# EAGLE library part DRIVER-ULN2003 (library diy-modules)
7-Channel Darlington NPN Transistor Module based on ULN2003 chip More details available here: https://www.elecrow.com/wiki/index.php?title=ULN2003_Stepper_Motor_Driver ULN2003 datasheet available here: http://www.ti.com/lit/ds/slrs027o/slrs027o.pdf Click here to find device on ebay.com Note: There are many variants. Search for the proper version.
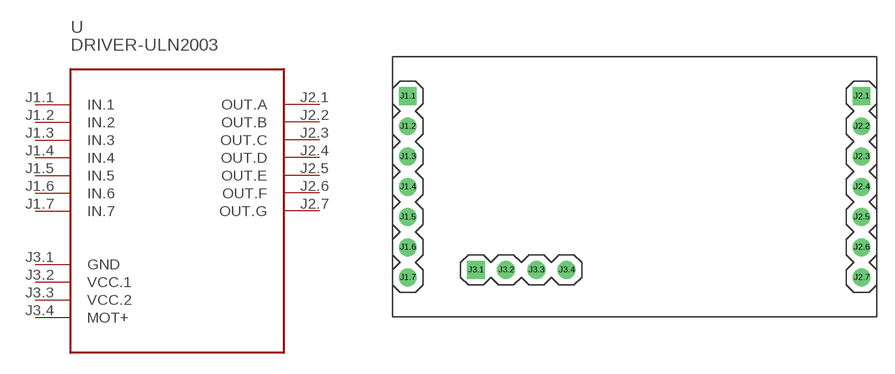
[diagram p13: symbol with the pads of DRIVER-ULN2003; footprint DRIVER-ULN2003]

Designator prefix -

## DRIVER-ULN2003  [DRIVER-ULN2003]
J1.1  IN.1
J1.2  IN.2
J1.3  IN.3
J1.4  IN.4
J1.5  IN.5
J1.6  IN.6
J1.7  IN.7
J2.1  OUT.A
J2.2  OUT.B
J2.3  OUT.C
J2.4  OUT.D
J2.5  OUT.E
J2.6  OUT.F
J2.7  OUT.G
J3.1  GND  pwr
J3.2  VCC.1  pwr
J3.3  VCC.2
J3.4  MOT+

## Footprint DRIVER-ULN2003 (pad centres in mm)
7-Channel Darlington NPN Transistor Module based on ULN2003 chip
drill 1 square: J1.1 -19.05,7.62; J2.1 19.05,7.62; J3.1 -13.335,-6.985
drill 1: J1.2 -19.05,5.08; J1.3 -19.05,2.54; J1.4 -19.05,0; J1.5 -19.05,-2.54; J1.6 -19.05,-5.08; J1.7 -19.05,-7.62; J2.2 19.05,5.08; J2.3 19.05,2.54; J2.4 19.05,0; J2.5 19.05,-2.54; J2.6 19.05,-5.08; J2.7 19.05,-7.62; J3.2 -10.795,-6.985; J3.3 -8.255,-6.985; J3.4 -5.715,-6.985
